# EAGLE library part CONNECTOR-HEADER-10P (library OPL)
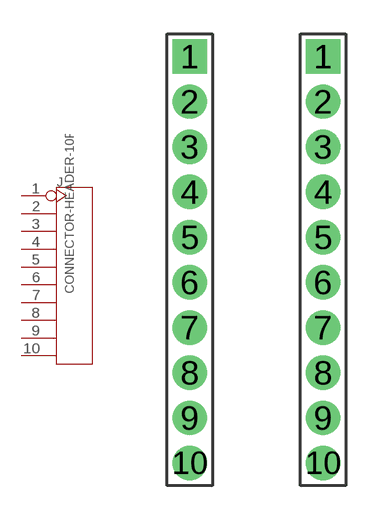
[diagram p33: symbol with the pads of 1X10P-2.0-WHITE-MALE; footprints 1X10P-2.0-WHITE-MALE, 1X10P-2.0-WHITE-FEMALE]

Designator prefix J

## CONNECTOR-HEADER-10P-320020018  [1X10P-2.0-WHITE-MALE]
1  1
2  2
3  3
4  4
5  5
6  6
7  7
8  8
9  9
10  10

## CONNECTOR-HEADER-10P-320030020  [1X10P-2.0-WHITE-FEMALE]
Pads as for 1X10P-2.0-WHITE-MALE

## CONNECTOR-HEADER-10P-3460510P1  [1X10P-2.0-4.3-BLUE-FEMALE]
Pads as for 1X10P-2.0-WHITE-MALE

## CONNECTOR-HEADER-10P-320030001  [1X10P-2.54-8.5--BLUE-FEMALE]
Pads as for 1X10P-2.0-WHITE-MALE

## CONNECTOR-HEADER-10P-320030039  [1X10P-2.54-8.5-BLACK-FEMALE]
Pads as for 1X10P-2.0-WHITE-MALE

## Footprint 1X10P-2.0-WHITE-MALE (pad centres in mm)
drill 0.813 pad 1.524 square: 1 0,9
drill 0.813 pad 1.524: 2 0,7; 3 0,5; 4 0,3; 5 0,1; 6 0,-1; 7 0,-3; 8 0,-5; 9 0,-7; 10 0,-9

## Footprint 1X10P-2.0-WHITE-FEMALE (pad centres in mm)
drill 0.813 pad 1.524 square: 1 0,9
drill 0.813 pad 1.524: 2 0,7; 3 0,5; 4 0,3; 5 0,1; 6 0,-1; 7 0,-3; 8 0,-5; 9 0,-7; 10 0,-9

## Footprint 1X10P-2.0-4.3-BLUE-FEMALE (pad centres in mm)
drill 0.813 pad 1.524 square: 1 0,9
drill 0.813 pad 1.524: 2 0,7; 3 0,5; 4 0,3; 5 0,1; 6 0,-1; 7 0,-3; 8 0,-5; 9 0,-7; 10 0,-9

## Footprint 1X10P-2.54-8.5--BLUE-FEMALE (pad centres in mm)
drill 0.889 pad 1.651 square: 1 0,11.43
drill 0.889 pad 1.651: 2 0,8.89; 3 0,6.35; 4 0,3.81; 5 0,1.27; 6 0,-1.27; 7 0,-3.81; 8 0,-6.35; 9 0,-8.89; 10 0,-11.43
